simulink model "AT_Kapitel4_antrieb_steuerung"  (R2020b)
settings: Solver=ode15s  StartTime=0.0  StopTime=60.0  RelTol=1e-3  EnableMultiTasking=on
InitFcn:
  | parameter
libraries: cstblocks x1

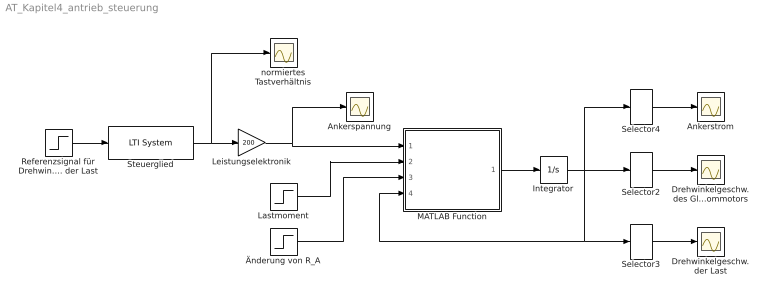
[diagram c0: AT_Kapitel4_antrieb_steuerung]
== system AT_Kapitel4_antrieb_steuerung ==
  Ankerspannung : Scope
  Ankerstrom : Scope
  Drehwinkelgeschw. der Last : Scope
  Drehwinkelgeschw. des Gleichstrommotors : Scope
  Integrator : Integrator  InitialCondition=zeros(5,1)
  Lastmoment : Step  Time=20  SampleTime=0
  Leistungselektronik : Gain  Gain=200  SaturateOnIntegerOverflow=on
  MATLAB Function : MATLAB Function  TreatAsAtomicUnit=on
  Referenzsignal für Drehwinkelgeschw. der Last : Step  Time=10  Before=100  After=-100  SampleTime=0
  Selector2 : Selector  InputPortWidth=5  IndexOptions=Index vector (dialog)  Indices=[3]  OutputSizes=1
  Selector3 : Selector  InputPortWidth=5  IndexOptions=Index vector (dialog)  Indices=[5]  OutputSizes=1
  Selector4 : Selector  InputPortWidth=5  IndexOptions=Index vector (dialog)  Indices=[1]  OutputSizes=1
  Steuerglied : cstblocks/LTI System  sys=R1  IC=[]
  normiertes Tastverhältnis : Scope
  Änderung von R_A : Step  Time=40  Before=1  After=1.4  SampleTime=0
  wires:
  Referenzsignal für Drehwinkelgeschw. der Last/1 -> Steuerglied/1
  Lastmoment/1 -> MATLAB Function/2(ML)
  Steuerglied/1 -> Leistungselektronik/1, normiertes Tastverhältnis/1
  Leistungselektronik/1 -> MATLAB Function/1(uA), Ankerspannung/1
  Änderung von R_A/1 -> MATLAB Function/3(kRA)
  MATLAB Function/1(dx) -> Integrator/1
  Integrator/1 -> Selector2/1, MATLAB Function/4(x), Selector3/1, Selector4/1
  Selector3/1 -> Drehwinkelgeschw. der Last/1
  Selector2/1 -> Drehwinkelgeschw. des Gleichstrommotors/1
  Selector4/1 -> Ankerstrom/1

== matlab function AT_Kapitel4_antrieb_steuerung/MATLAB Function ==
function dx = Antrieb(uA,ML,kRA,x,par)

% define parameters
RA    = par.R_A;
LA    = par.L_A;
kA    = par.k_A;
thetaG = par.theta_G;
thetaL = par.theta_L;
cT    = par.c_T;
dT    = par.d_T;

% define x, y, u, p for better code readability
iA=x(1);
phi1=x(2);
omega1=x(3);
phi2=x(4);
omega2=x(5);

% ODE's
dx=zeros(5,1);
dx(1)=1/LA*(-RA*iA*kRA-kA*omega1+uA);
dx(2)=omega1;
dx(3)=1/thetaG*(kA*iA-cT*(phi1-phi2)-dT*(omega1-omega2));
dx(4)=omega2;
dx(5)=1/thetaL*(cT*(phi1-phi2)+dT*(omega1-omega2)-ML);

end
